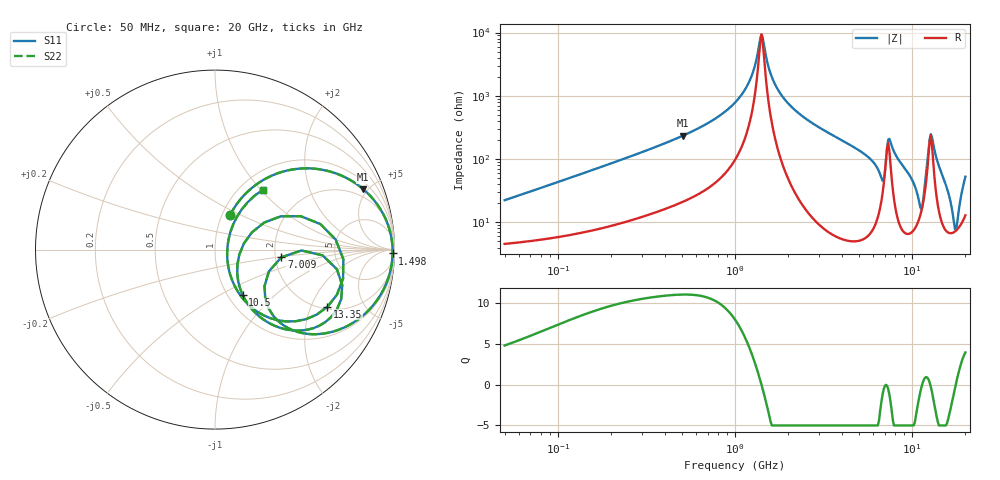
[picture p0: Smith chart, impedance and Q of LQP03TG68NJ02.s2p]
!Murata Part Number: LQP03TG68NJ02
!These Parameters are Measured in Series Mode Connection
!  o--[Z]--o
!Port1  Port2
!  o-------o
!Freq. Start=50[MHz] Stop=20[GHz], 401[Steps]
# Hz S RI R 50
!Freq.(Hz) S11(Real) S11(Imag) S21(Real) S21(Imag) S12(Real) S12(Imag) S22(Real) S22(Imag)
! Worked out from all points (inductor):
!   401 points, 50 MHz to 20 GHz, reference 50 ohm
!   read as one part in series: L = 69 nH near 51.52 MHz
!   highest Q = 11 at 509.6 MHz (marker M1), where L = 73.2 nH
!   self-resonance near 1.39 GHz
!   S11 on the Smith chart (normalised r, x): 50 MHz: 1.09, +0.44; 1.498 GHz: 35, -75; 7.009 GHz: 2.16, -0.21; 10.5 GHz: 1.17, -0.65; 13.35 GHz: 2.10, -2.64; 20 GHz: 1.26, +1.02
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5e7  0.0837 0.1918  0.9163 -0.1918  0.9163 -0.1918  0.0837 0.1918
1.364002e8  0.2785 0.3933  0.7215 -0.3933  0.7215 -0.3933  0.2785 0.3933
3.721004e8  0.7094 0.4102  0.2906 -0.4102  0.2906 -0.4102  0.7094 0.4102
5.096456e8  0.8259 0.3367  0.1741 -0.3367  0.1741 -0.3367  0.8259 0.3367
1e9  0.9692 0.1212  0.0308 -0.1212  0.0308 -0.1212  0.9692 0.1212
1.214974e9  0.9847 0.0532  0.0153 -0.0532  0.0153 -0.0532  0.9847 0.0532
1.390315e9  0.9892 0.00534  0.0108 -0.00534  0.0108 -0.00534  0.9892 0.00534
1.498439e9  0.9895 -0.0216  0.0105 0.0216  0.0105 0.0216  0.9895 -0.0216
1.820564e9  0.9825 -0.0928  0.0175 0.0928  0.0175 0.0928  0.9825 -0.0928
2.728004e9  0.9254 -0.2472  0.0746 0.2472  0.0746 0.2472  0.9254 -0.2472
5.769027e9  0.5105 -0.469  0.4895 0.469  0.4895 0.469  0.5105 -0.469
7.009217e9  0.3703 -0.0428  0.6297 0.0428  0.6297 0.0428  0.3703 -0.0428
7.442007e9  0.709 -0.199  0.291 0.199  0.291 0.199  0.709 -0.199
8.389408e9  0.4889 -0.45  0.5111 0.45  0.5111 0.45  0.4889 -0.45
1.050288e10  0.1545 -0.2537  0.8455 0.2537  0.8455 0.2537  0.1545 -0.2537
1.131968e10  0.136 -0.0261  0.864 0.0261  0.864 0.0261  0.136 -0.0261
1.201863e10  0.3668 0.1856  0.6332 -0.1856  0.6332 -0.1856  0.3668 0.1856
1.276073e10  0.715 -0.0533  0.285 0.0533  0.285 0.0533  0.715 -0.0533
1.334722e10  0.6267 -0.3181  0.3733 0.3181  0.3733 0.3181  0.6267 -0.3181
1.550395e10  0.1749 -0.2954  0.8251 0.2954  0.8251 0.2954  0.1749 -0.2954
1.747767e10  0.0676 -0.0249  0.9324 0.0249  0.9324 0.0249  0.0676 -0.0249
2e10  0.2651 0.3327  0.7349 -0.3327  0.7349 -0.3327  0.2651 0.3327
